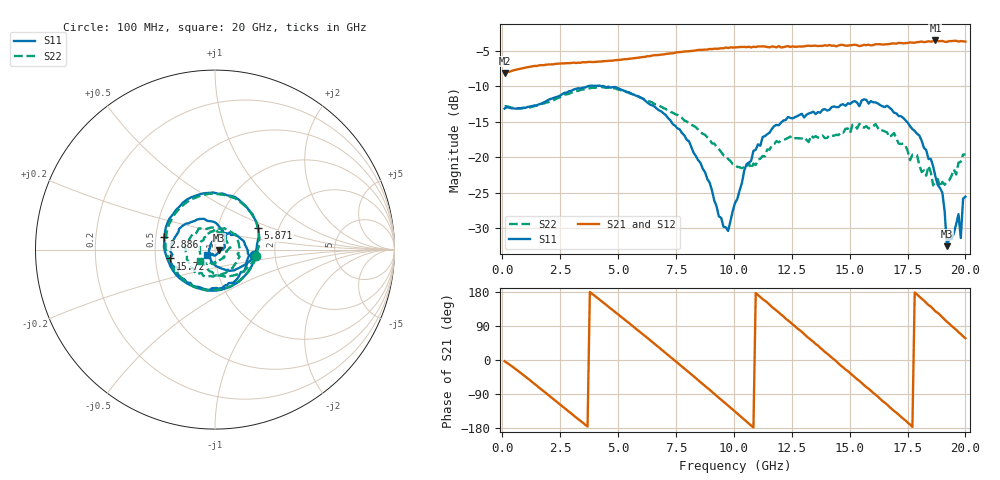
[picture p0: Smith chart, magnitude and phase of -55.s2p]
!Agilent Technologies,N5230C,MY49001569,A.09.33.09
!Agilent N5230C: A.09.33.09
!Date: Monday, July 27, 2015 12:42:44
!Correction: S11(Full 2 Port(1,2))
!S21(Full 2 Port(1,2))
!S12(Full 2 Port(1,2))
!S22(Full 2 Port(1,2))
!S2P File: Measurements: S11, S21, S12, S22:
# Hz S  dB  R 50
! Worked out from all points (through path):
!   201 points, 100 MHz to 20 GHz, reference 50 ohm
!   highest |S21| = -3.53 dB at 18.71 GHz (marker M1); lowest = -8.1 dB at 100 MHz (marker M2)
!   group delay of S21, straight-line fit = 143 ps
!   lowest |S11| = -32.5 dB at 19.2 GHz (marker M3), VSWR 1.05, Z = 52.4 - j0.229 ohm
!   |S11| at or under -10 dB: start of sweep to 3.674 GHz; 4.408 GHz to end of sweep
!   |S22| runs from -24.1 to -10.1 dB; largest |S21 - S12| = 0.03
!   S11 on the Smith chart (normalised r, x): 100 MHz: 1.55, -0.11; 2.886 GHz: 0.55, +0.08; 5.871 GHz: 1.57, +0.41; 15.72 GHz: 0.60, -0.06; 20 GHz: 0.91, -0.05
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1e8  -13.12 -8.5  -8.10 -3.2  -8.07 -3.4  -12.76 -8.7
1.692e9  -12.42 -122.1  -7.00 -77.8  -7.04 -77.9  -12.44 -120.6
2.886e9  -10.68 166.3  -6.72 -136.7  -6.73 -137.1  -11.04 166.1
3.483e9  -10.17 134.4  -6.58 -165.6  -6.64 -166.1  -10.44 134.9
5.871e9  -11.40 26.8  -5.96 77.7  -5.97 77.2  -11.41 27.6
6.7665e9  -13.36 -10.4  -5.58 33.0  -5.53 32.6  -12.70 -8.3
7.7615e9  -16.57 -51.9  -5.14 -17.2  -5.19 -17.9  -14.44 -45.7
8.7565e9  -22.09 -98.6  -4.81 -68.5  -4.83 -69.4  -16.81 -86.4
9.5525e9  -29.78 177.0  -4.64 -110.0  -4.61 -110.7  -19.69 -124.5
1.005e10  -26.44 107.6  -4.52 -136.2  -4.50 -137.1  -21.06 -158.3
1.1443e10  -16.73 31.8  -4.44 151.8  -4.41 149.9  -18.88 90.8
1.23385e10  -14.30 -9.5  -4.33 104.4  -4.46 104.4  -17.25 39.1
1.3433e10  -13.56 -61.5  -4.27 48.2  -4.34 46.4  -17.21 -23.6
1.4627e10  -12.58 -119.0  -4.15 -15.0  -4.23 -15.7  -16.42 -94.0
1.57215e10  -11.89 -168.8  -4.19 -71.6  -4.21 -72.0  -15.60 -160.4
1.67165e10  -12.98 144.0  -4.03 -123.6  -4.01 -123.6  -17.16 141.0
1.77115e10  -16.01 96.8  -3.84 -176.7  -3.85 -178.1  -19.62 69.3
1.87065e10  -22.72 44.9  -3.53 128.3  -3.75 128.5  -23.29 -16.1
1.9005e10  -24.97 13.7  -3.60 112.9  -3.62 111.1  -23.45 -41.6
1.9204e10  -32.50 -5.3  -3.74 100.8  -3.65 101.1  -23.44 -72.8
1.9801e10  -31.35 -115.0  -3.61 68.5  -3.75 66.7  -20.61 -132.9
2e10  -25.53 -148.5  -3.69 57.4  -3.69 56.6  -19.59 -142.8
